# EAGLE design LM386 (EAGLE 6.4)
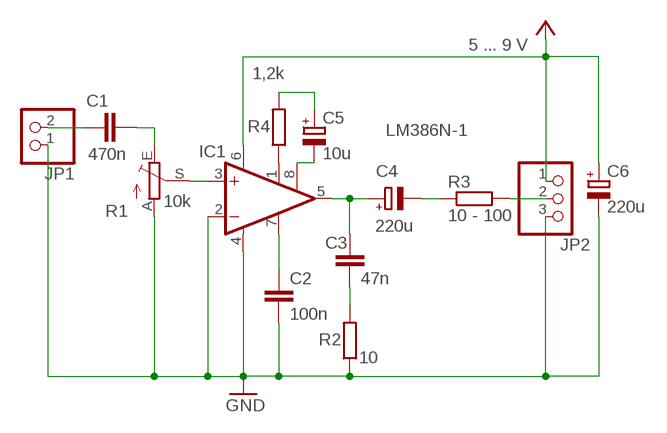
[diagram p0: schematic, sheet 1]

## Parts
C1  470n  C-EU025-025X050  [C025-025X050]
C2  100n  C-EU025-025X050  [C025-025X050]
C3  47n  C-EU025-025X050  [C025-025X050]
C4  220u  CPOL-EUE5-5  [E5-5]
C5  10u  CPOL-EUE5-5  [E5-5]
C6  220u  CPOL-EUE5-5  [E5-5]
IC1  LM386N-1  [DIL08]
JP1  PINHD-1X2  [1X02]
JP2  PINHD-1X3  [1X03]
R1  10k  TRIM_EU-LI10  [LI10]
R2  10  R-EU_0207/10  [0207/10]
R3  10 - 100  R-EU_0207/10  [0207/10]
R4  1,2k  R-EU_0207/10  [0207/10]

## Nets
GND: C2.2 C6.- IC1.2(-IN) IC1.4(GND) JP1.1 JP2.3 R1.A R2.1
N$1: C1.1 JP1.2
N$2: C1.2 R1.E
N$3: IC1.3(+IN) R1.S
N$4: C2.1 IC1.7(BYPASS)
N$5: C3.2 R2.2
N$6: C3.1 C4.+ IC1.5(OUT)
N$7: C4.- R3.1
N$8: JP2.2 R3.2
N$9: IC1.1(GAIN) R4.1
N$11: C5.+ R4.2
N$12: C5.- IC1.8(GAIN)
VCC: C6.+ IC1.6(VS) JP2.1 ; supply symbol labelled 5 ... 9 V

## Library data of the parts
C1-C3 = rcl:C-EU: CAPACITOR, European symbol
C4-C6 = rcl:CPOL-EU: POLARIZED CAPACITOR, European symbol
IC1 = linear:LM386?-*: Low Voltage Audio Power Amplifier Source: http://cache.national.com/ds/LM/LM386.pdf
JP1 = pinhead:PINHD-1X2: PIN HEADER
JP2 = pinhead:PINHD-1X3: PIN HEADER
R1 = pot:TRIM_EU-: POTENTIOMETER
R2-R4 = rcl:R-EU_: RESISTOR, European symbol

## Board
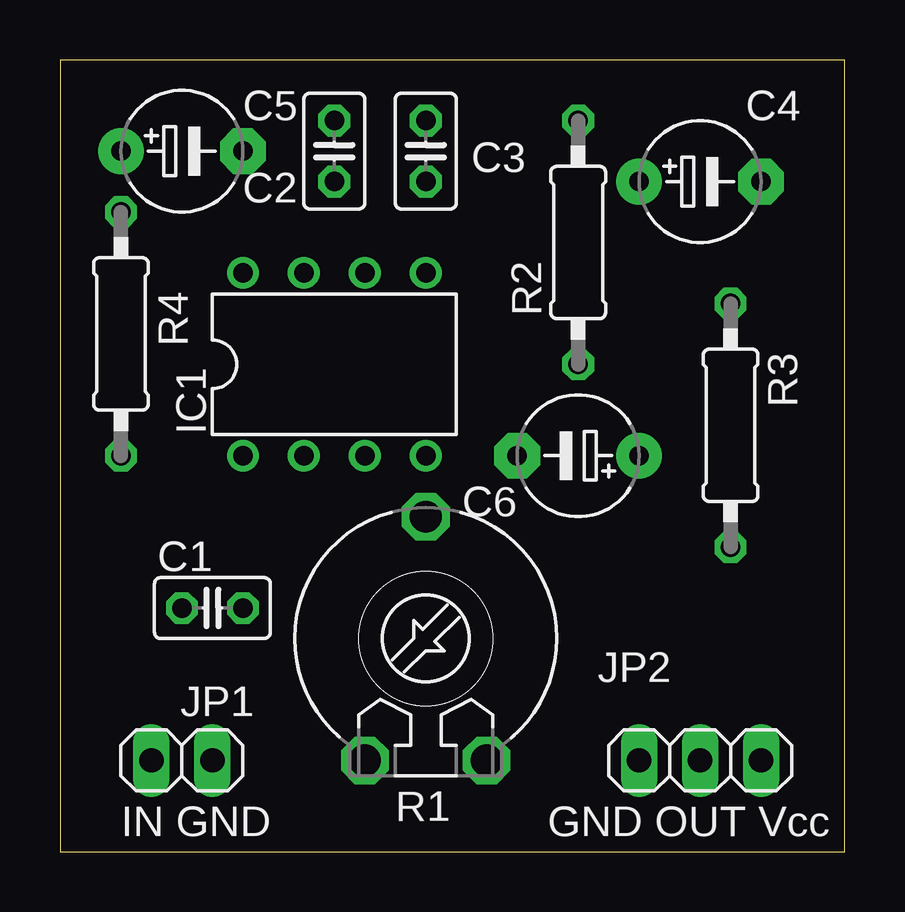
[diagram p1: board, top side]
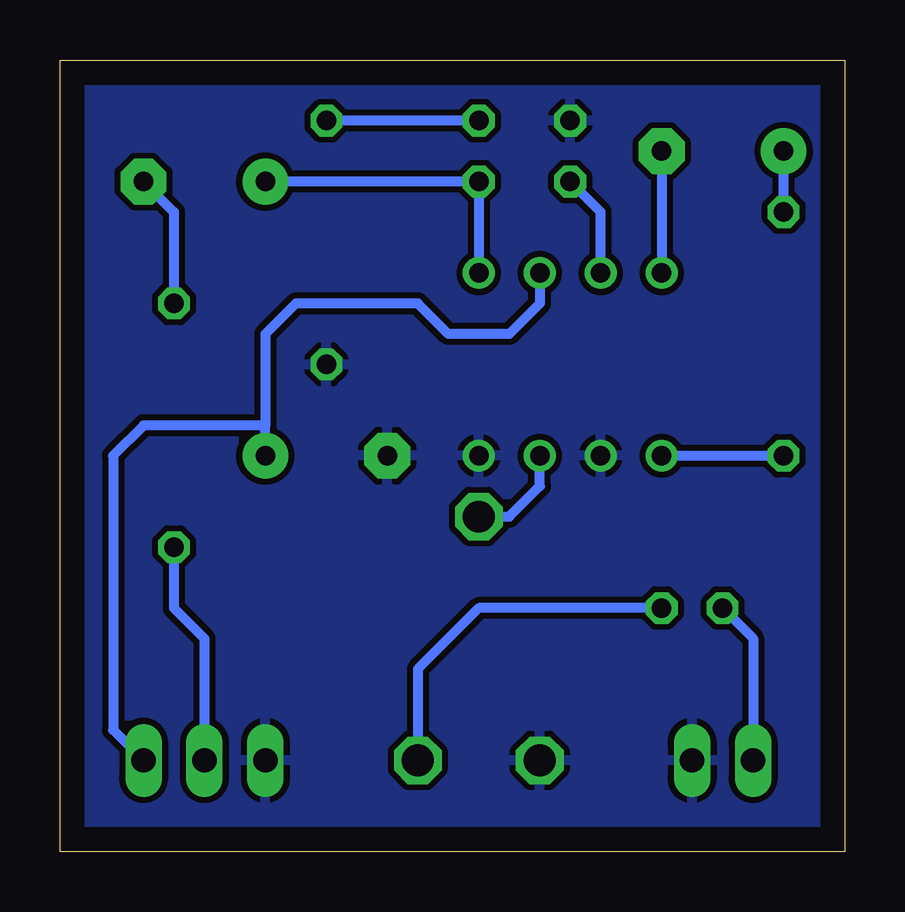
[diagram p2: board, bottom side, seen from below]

Size 32.69 x 33.01 mm. Coordinates in mm from the lower left corner, seen from the top.
Outline: 0,0 32.69,0 32.69,33.01 0,33.01 0,0
Copper layers (1*16): Top 0.035mm / dielectric 1.5mm / Bottom 0.035mm
Design rules "default": minimum track width 10mil, minimum drill 24mil, track to track 8mil, track to pad 8mil, pad to pad 8mil, via to via 8mil, smd to smd 8mil, copper to edge 40mil, drill to drill 8mil, minimum pad ring 10mil, minimum via ring 8mil, stop-mask expansion 4mil, vias tented up to drill 0mil, thermal gap 10mil

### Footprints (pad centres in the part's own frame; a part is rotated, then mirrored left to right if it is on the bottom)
C025-025X050 = drill 0.813 octagon: 1 -1.27,0; 2 1.27,0
E5-5 = drill 0.813 pad 1.905: + -2.54,0 | drill 0.813 pad 1.905 octagon: - 2.54,0
DIL08 = drill 0.813 pad 1.27: 1 -3.81,-3.81; 2 -1.27,-3.81; 3 1.27,-3.81; 4 3.81,-3.81; 5 3.81,3.81; 6 1.27,3.81; 7 -1.27,3.81; 8 -3.81,3.81
1X02 = drill 1.016 long: 1 -1.27,0; 2 1.27,0
1X03 = drill 1.016 long: 1 -2.54,0; 2 0,0; 3 2.54,0
LI10 = drill 1.321 octagon: A -2.54,-5.08; E 2.54,-5.08; S 0,5.08
0207/10 = drill 0.813 octagon: 1 -5.08,0; 2 5.08,0

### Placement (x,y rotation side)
C1  6.35,10.16 0 top
C2  11.43,29.21 90 top
C3  15.24,29.21 90 top
C4  26.67,27.94 0 top
C5  5.08,29.21 0 top
C6  21.59,16.51 180 top
IC1  11.43,20.32 0 top
JP1  5.08,3.81 180 top
JP2  26.67,3.81 180 top
R1  15.24,8.89 0 top
R2  21.59,25.4 90 top
R3  27.94,17.78 270 top
R4  2.54,21.59 90 top

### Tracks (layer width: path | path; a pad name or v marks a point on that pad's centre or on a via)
GND
  pour Bottom (isolate 0.254): 0,33.02 33.02,33.02 33.02,0 0,0
N$1
  Bottom 0.406: C1.1 3.81,8.89 JP1.2
N$2
  Bottom 0.406: C1.2 15.24,10.16 17.78,7.62 R1.E
N$3
  Bottom 0.406: R1.S 13.97,13.97 12.7,15.24 IC1.3
N$4
  Bottom 0.406: IC1.7 10.16,26.67 C2.1
N$5
  Bottom 0.406: C3.2 R2.2
N$6
  Bottom 0.406: IC1.5 C3.1 C4.+
N$7
  Bottom 0.406: C4.- 27.94,26.67 R3.1
N$8
  Bottom 0.406: R3.2 27.94,10.16 26.67,8.89 JP2.2
N$9
  Bottom 0.406: IC1.1 R4.1
N$11
  Bottom 0.406: R4.2 C5.+
N$12
  Bottom 0.406: C5.- IC1.8
VCC
  Bottom 0.406: IC1.6 12.7,22.86 13.97,21.59 16.51,21.59 17.78,22.86 22.86,22.86 24.13,21.59 24.13,17.78 | C6.+ 24.13,17.78 | 24.13,17.78 29.21,17.78 30.48,16.51 30.48,5.08 JP2.1

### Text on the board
tNames: IN GND | GND OUT Vcc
